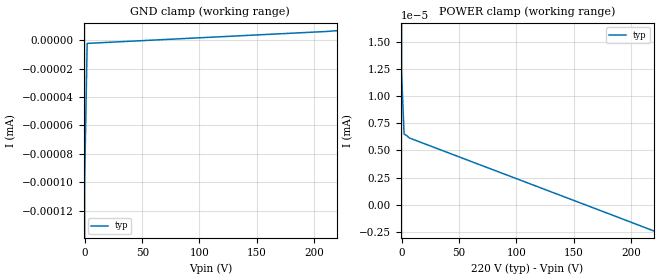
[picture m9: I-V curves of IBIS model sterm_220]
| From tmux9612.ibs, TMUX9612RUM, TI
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| sterm_220
[Model]   sterm_220
Model_type   Terminator
|   typ   min   max
C_comp   1.008417e-11   NA   NA
[Voltage Range]   220   NA   NA
[Temperature Range]   27   NA   NA
[Power Clamp Reference]   220   NA   NA
[GND Clamp Reference]   0   NA   NA
[GND Clamp]
|   Voltage   I(typ)   I(min)   I(max)
-5V       -2.415A    NA         NA
-2.727V   -784mA     NA         NA
-454.5mV  -102.8nA   NA         NA
1.818V    -2.337nA   NA         NA
220V      6.559nA    NA         NA
[POWER Clamp]
|   Voltage   I(typ)   I(min)   I(max)
-5V       1.055A     NA         NA
-2.727V   432.7mA    NA         NA
-455mV    12.37nA    NA         NA
1.818V    6.511nA    NA         NA
6.364V    6.155nA    NA         NA
220V      -2.411nA   NA         NA
